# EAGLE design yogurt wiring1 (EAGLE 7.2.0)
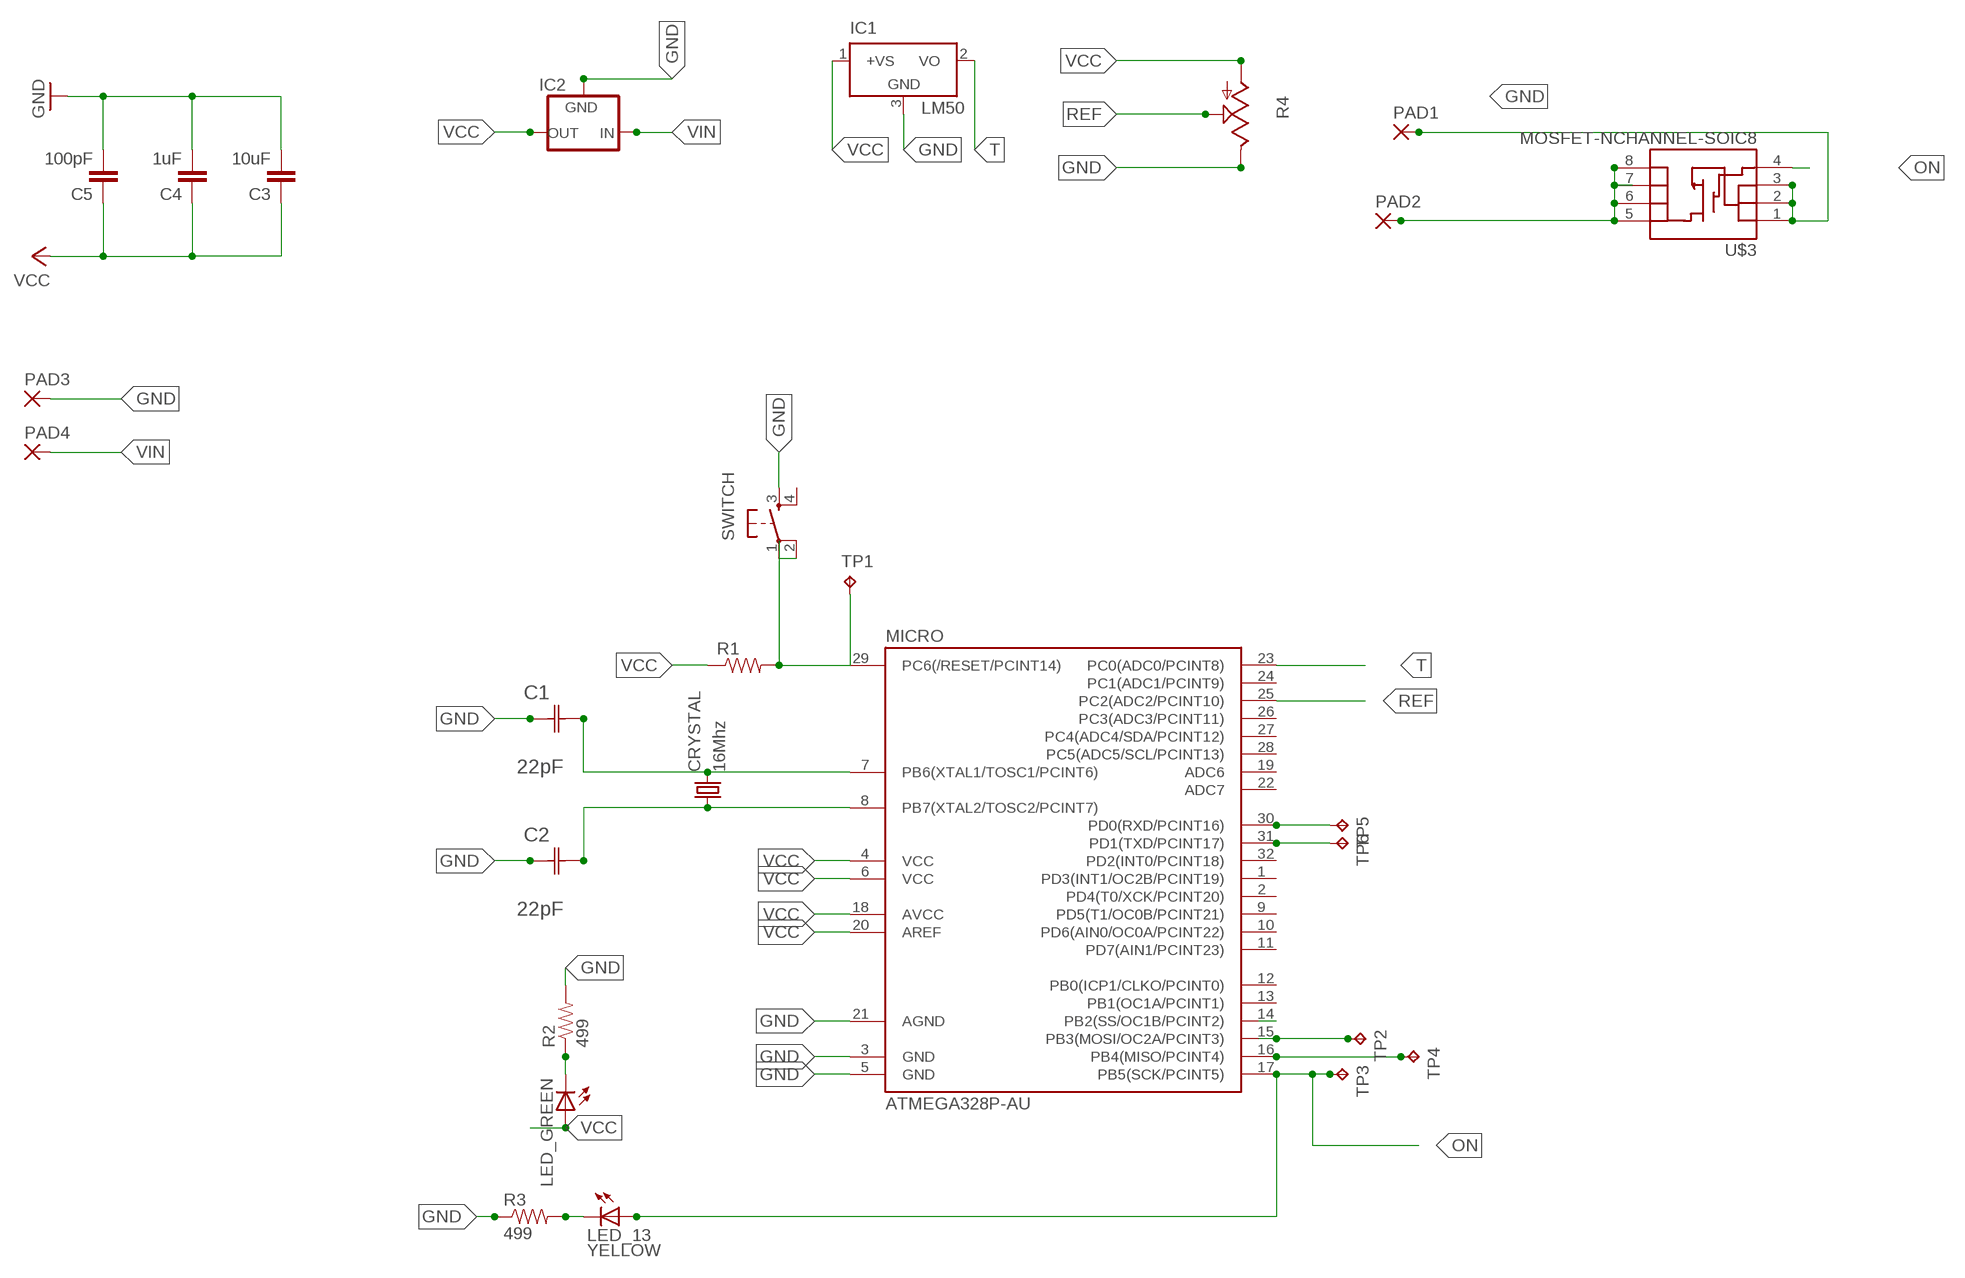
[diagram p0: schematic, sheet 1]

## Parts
C1  22pF  0612ZC225MAT2A  [CAPC3216X178N]
C2  22pF  0612ZC225MAT2A  [CAPC3216X178N]
C3  10uF  CAP1206  [1206]
C4  1uF  CAP1206  [1206]
C5  100pF  CAP1206  [1206]
CRYSTAL  16Mhz  CSM-7X-DU  [CSM-7X-DU]
IC1  LM50  [SOT23]
IC2  V_REG_78XXSIDE  [78XXL]
LED_13  YELLOW  LED1206  [1206]
LED_GREEN  LED1206  [1206]
MICRO  ATMEGA328P-AU  ATMEGA48/88/168-AU  [TQFP32-08]
PAD1  SMD5  [SMD2,54-5,08]
PAD2  SMD5  [SMD2,54-5,08]
PAD3  SMD5  [SMD2,54-5,08]
PAD4  SMD5  [SMD2,54-5,08]
R1  RESISTOR1206  [1206]
R2  499  RESISTOR1206  [1206]
R3  499  RESISTOR1206  [1206]
R4  TRIM_US-SM-42/43X  [SM-42/43X]
SWITCH  6MM_SWITCH6MM_SWITCH  [6MM_SWITCH]
TP1  TPPAD1-17Y  [P1-17Y]
TP2  TPPAD1-17Y  [P1-17Y]
TP3  TPPAD1-17Y  [P1-17Y]
TP4  TPPAD1-17Y  [P1-17Y]
TP5  TPPAD1-17Y  [P1-17Y]
TP6  TPPAD1-17Y  [P1-17Y]
U$3  MOSFET-NCHANNEL-SOIC8  [SO08]

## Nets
GND: C1.1(C1) C2.1(C1) C3.2 C4.2 C5.2 IC1.3(GND) IC2.GND MICRO.3(GND) MICRO.5(GND) MICRO.21(AGND) PAD1.1(P) PAD3.1(P) R2.2 R3.1 R4.3(E) SWITCH.3(S) U$3.1(S) U$3.2(S) U$3.3(S)
N$2: C1.2(C2) CRYSTAL.2 MICRO.7(PB6(XTAL1/TOSC1/PCINT6))
N$4: MICRO.29(PC6(/RESET/PCINT14)) R1.2 SWITCH.1(P) SWITCH.2(P1) TP1.TP
N$5: MICRO.15(PB3(MOSI/OC2A/PCINT3)) TP2.TP
N$6: MICRO.14(PB2(SS/OC1B/PCINT2))
N$7: MICRO.31(PD1(TXD/PCINT17)) TP6.TP
N$8: MICRO.30(PD0(RXD/PCINT16)) TP5.TP
N$9: C2.2(C2) CRYSTAL.1 MICRO.8(PB7(XTAL2/TOSC2/PCINT7))
N$11: MICRO.16(PB4(MISO/PCINT4)) TP4.TP
N$26: LED_GREEN.2(C) R2.1
N$27: LED_13.2(C) R3.2
N$35: PAD2.1(P) U$3.5(D) U$3.6(D) U$3.7(D) U$3.8(D)
ON: LED_13.1(A) MICRO.17(PB5(SCK/PCINT5)) TP3.TP U$3.4(G)
REF: MICRO.25(PC2(ADC2/PCINT10)) R4.2(S)
T: IC1.2(VO) MICRO.23(PC0(ADC0/PCINT8))
VCC: C3.1 C4.1 C5.1 IC1.1(+VS) IC2.OUT LED_GREEN.1(A) MICRO.4(VCC) MICRO.6(VCC) MICRO.18(AVCC) MICRO.20(AREF) R1.1 R4.1(A)
VIN: IC2.IN PAD4.1(P)
Unconnected: MICRO.1(PD3(INT1/OC2B/PCINT19)) MICRO.2(PD4(T0/XCK/PCINT20)) MICRO.9(PD5(T1/OC0B/PCINT21)) MICRO.10(PD6(AIN0/OC0A/PCINT22)) MICRO.11(PD7(AIN1/PCINT23)) MICRO.12(PB0(ICP1/CLKO/PCINT0)) MICRO.13(PB1(OC1A/PCINT1)) MICRO.19(ADC6) MICRO.22(ADC7) MICRO.24(PC1(ADC1/PCINT9)) MICRO.26(PC3(ADC3/PCINT11)) MICRO.27(PC4(ADC4/SDA/PCINT12)) MICRO.28(PC5(ADC5/SCL/PCINT13)) MICRO.32(PD2(INT0/PCINT18)) SWITCH.4(S1)

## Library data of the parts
C1 C2 = AVX_By_element14_Batch_1:0612ZC225MAT2A: Capacitor 1206; MPN: 0612ZC225MAT2A; OC_FARNELL: -; OC_NEWARK: 12N3209; SUPPLIER: AVX; TOLERANCE: ±20%; VALUE: 2.2µF; VOLTAGERATING: 10V
C3-C5 = 01_SparkFun:CAP: Capacitor
CRYSTAL = 01_FAB_Hello:CSM-7X-DU: SMD CRYSTAL; OC_FARNELL: unknown; OC_NEWARK: unknown
IC1 = linear:LM50: SOT-23 Single-Supply Centigrade Temperature Sensor Vout = (10mV/°C x Temp °C) +5mmmV Source: http://cache.national.com/ds/LM/LM50.pdf
IC2 = 01_SparkFun:V_REG_78XX: Voltage Regulator Standard 7805 5V regulator. IGO (Input Ground Output). Spark Fun Electronics SKU : COM-00107
LED_13 LED_GREEN = 01_FAB_Hello:LED
MICRO = atmega8:ATMEGA48/88/168
PAD1-PAD4 = wirepad:SMD5: SMD PAD
R1-R3 = 01_SparkFun:RESISTOR: Resistor
R4 = pot:TRIM_US-: POTENTIOMETER
SWITCH = 01_FAB_Hello:6MM_SWITCH: OMRON SWITCH
TP1-TP6 = testpad:TP: Test pad
U$3 = 01_SparkFun:MOSFET-NCHANNEL-SOIC8: N-Channel MOSFET IRF9410 and NDS8434 are common, SOIC-8 parts.

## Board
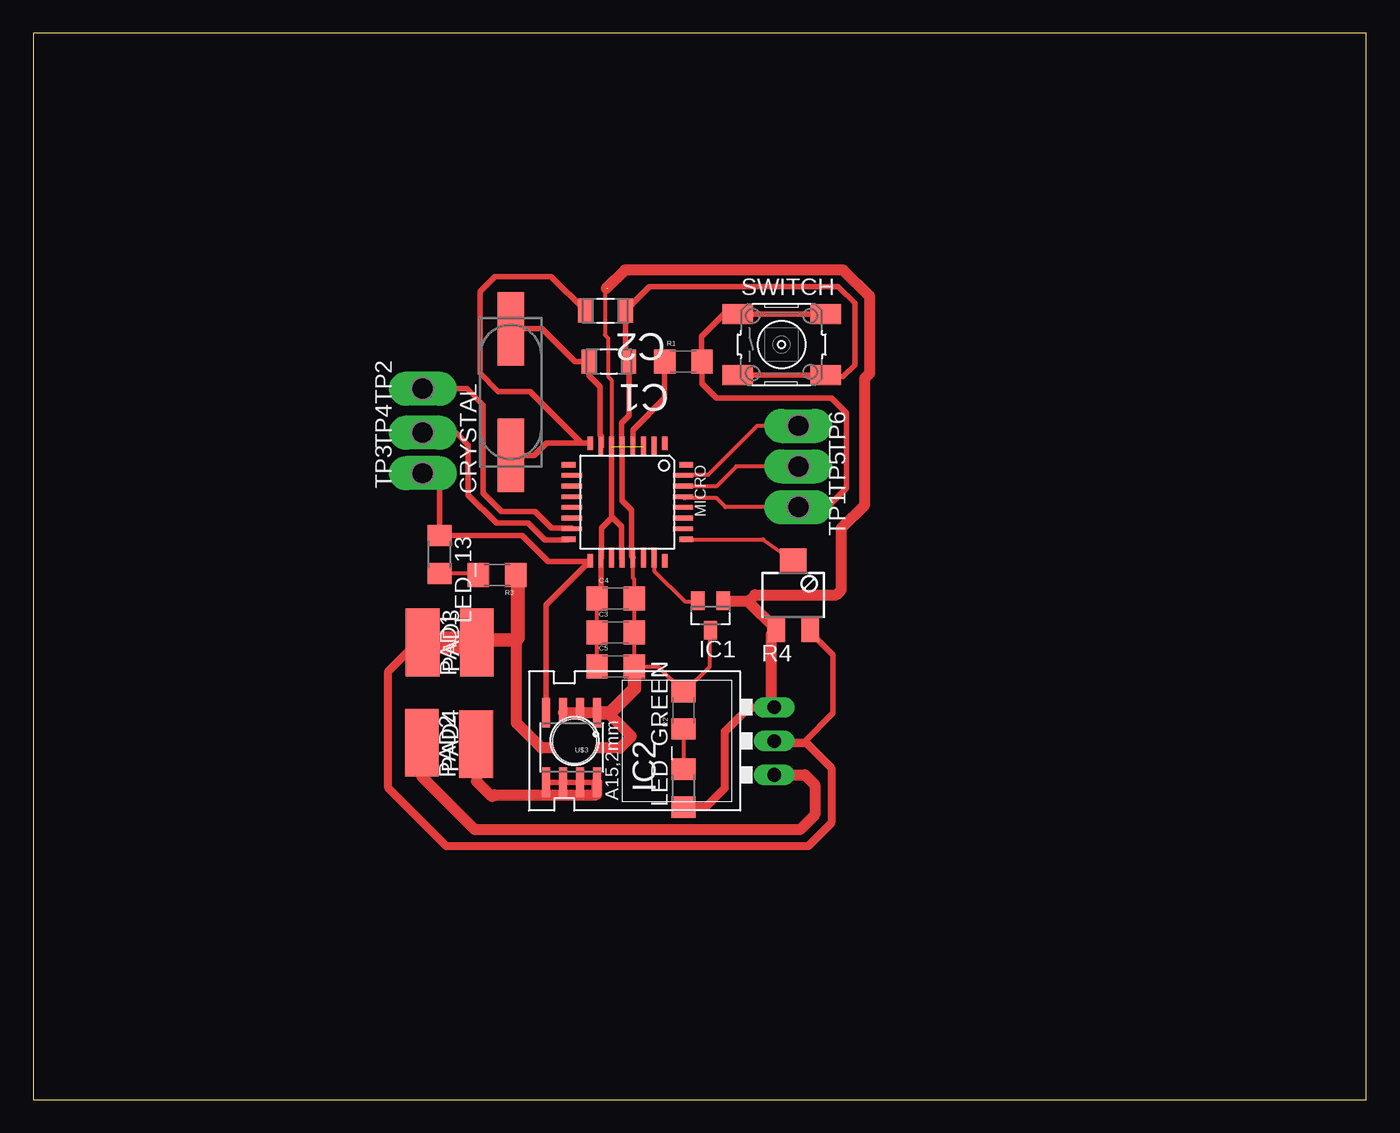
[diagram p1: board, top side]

Size 100 x 80 mm. Coordinates in mm from the lower left corner, seen from the top.
Outline: 0,0 100,0 100,80 0,80 0,0
Copper layers (1*16): Top 0.035mm / dielectric 1.5mm / Bottom 0.035mm
Design rules "default *": minimum track width 16mil, minimum drill 24mil, track to track 12mil, track to pad 12mil, pad to pad 12mil, via to via 12mil, smd to smd 12mil, copper to edge 40mil, drill to drill 8mil, minimum pad ring 10mil, minimum via ring 8mil, stop-mask expansion 4mil, vias tented up to drill 0mil, thermal gap 10mil

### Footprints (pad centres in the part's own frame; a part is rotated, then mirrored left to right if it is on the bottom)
CAPC3216X178N = smd 1.118 x 1.803: 1 -1.499,0; 2 1.499,0
1206 = smd 1.6 x 1.8: 1 -1.4,0; 2 1.4,0
CSM-7X-DU = smd 5.5 x 2: 1 -4.75,0; 2 4.75,0
SOT23 = smd 1 x 1.4: 1 -0.95,-1.1; 2 0.95,-1.1; 3 0,1.1
78XXL = drill 1.016 long: GND 0,-3.81; IN -2.54,-3.81; OUT 2.54,-3.81 | hole 3.302: 0,11.176
1206' = smd 1.6 x 1.803: 1 -1.422,0; 2 1.422,0
TQFP32-08 = smd 1.016 x 0.406: 1 -4.42,2.8; 8 -4.42,-2.8; 17 4.42,-2.8; 24 4.42,2.8 | smd 1.524 x 0.356: 2 -4.166,2; 3 -4.166,1.2; 4 -4.166,0.4; 5 -4.166,-0.4; 6 -4.166,-1.2; 7 -4.166,-2; 18 4.166,-2; 19 4.166,-1.2; 20 4.166,-0.4; 21 4.166,0.4; 22 4.166,1.2; 23 4.166,2 | smd 0.406 x 1.016: 9 -2.8,-4.42; 16 2.8,-4.42; 25 2.8,4.42; 32 -2.8,4.42 | smd 0.356 x 1.524: 10 -2,-4.166; 11 -1.2,-4.166; 12 -0.4,-4.166; 13 0.4,-4.166; 14 1.2,-4.166; 15 2,-4.166; 26 2,4.166; 27 1.2,4.166; 28 0.4,4.166; 29 -0.4,4.166; 30 -1.2,4.166; 31 -2,4.166
SMD2,54-5,08 = smd 2.54 x 5.08: 1 0,0
SM-42/43X = smd 1.3 x 1.9: 1 -1.27,-2.55; 3 1.27,-2.55 | smd 2 x 1.9: 2 0,2.55
6MM_SWITCH = smd 2.286 x 1.524: 1 -3.302,2.286; 2 3.302,2.286; 3 -3.302,-2.286; 4 3.302,-2.286
P1-17Y = drill 1.702 pad 2.121 long: TP 0,0
SO08 = smd 0.61 x 2.21: 1 -1.905,-2.616; 2 -0.635,-2.616; 3 0.635,-2.616; 4 1.905,-2.616; 5 1.905,2.616; 6 0.635,2.616; 7 -0.635,2.616; 8 -1.905,2.616

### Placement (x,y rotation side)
C1  43.18,55.37 180 top
C2  42.93,59.18 180 top
C3  43.69,35.05 0 top
C4  43.69,37.59 0 top
C5  43.69,32.51 0 top
CRYSTAL  35.81,53.09 90 top
IC1  50.8,36.32 180 top
IC2  51.78,26.9 90 top
LED_13  YELLOW  [1206']  30.48,40.89 270 top
LED_GREEN  [1206']  48.77,23.37 90 top
MICRO  44.58,44.83 270 top
PAD1  33.27,34.29 0 top
PAD2  33.21,26.66 0 top
PAD3  29.21,34.29 180 top
PAD4  29.15,26.78 180 top
R1  48.77,55.37 0 top
R2  48.77,29.21 90 top
R3  34.8,39.37 180 top
R4  57.02,37.84 0 top
SWITCH  56.13,56.64 0 top
TP1  57.4,44.45 270 top
TP2  29.21,53.34 90 top
TP3  29.21,46.99 90 top
TP4  29.21,50.04 90 top
TP5  57.4,47.5 270 top
TP6  57.4,50.55 270 top
U$3  40.39,26.42 180 top

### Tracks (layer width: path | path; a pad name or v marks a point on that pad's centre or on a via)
GND  (1 unrouted)
  Top 0.305: MICRO.21 45,40.64 45,39.12 45.09,39.04 C4.2 C3.2 C5.2 46.87,32.51 R2.2 48.86,30.61 50.75,32.5 50.75,35.17 IC1.3
  Top 0.406: MICRO.21 44.88,40.76 44.88,44.25 44.17,44.95 MICRO.5 44.12,49.05 44.12,50.75 44.68,51.3 C1.1 44.42,55.63 C2.1 46.24,61 60.38,61 61.62,59.75 61.62,55.12 60.75,54.25 59.5,54.25 59.39,54.36 SWITCH.3 | R4.3 58.29,35.09 60,33.38 60,29 57.88,26.88 55.61,26.88 IC2.GND | 36.25,39.32 36.38,39.32 36.38,38.25
  Top 0.61: U$3.3 U$3.2 U$3.1 | IC2.GND 55.74,26.75 58,26.75 59.88,24.88 59.88,20.75 58.12,19 31,19 26.62,23.38 26.62,32.12 28.79,34.29 PAD3.1
  Top 0.813: U$3.3 43.09,29.03 44.88,27.25 44,26.38 38.12,26.38 36.25,28.25 36.25,39.32 R3.1
  Top 1.016: PAD1.1 33.48,34.5 36.25,34.5 36.38,34.62 36.38,38.25 36.38,38.75 | C5.2 45.09,30.84 43.25,29 42.32,29 U$3.1
  Top 1.676: PAD3.1 PAD1.1
N$2
  Top 0.406: CRYSTAL.2 38.16,57.84 40.62,55.38 C1.2 41.68,54.32 42.5,53.5 42.5,49.88 42.62,49.75 42.62,49.05 MICRO.7
N$4
  Top 0.305: TP1.TP 51.92,44.45 51.25,45.12 48.84,45.12 MICRO.29
  Top 0.406: SWITCH.2 SWITCH.1 51.8,58.93 50.12,57.25 50.12,55.41 R1.2 50.17,53.71 51.25,52.62 59.88,52.62 61,51.5 61,45.88 59.5,44.38 57.48,44.38 TP1.TP
N$5
  Top 0.406: TP2.TP 32.53,53.34 33.75,52.12 33.75,45.5 35.12,44.12 37.62,44.12 38.88,42.88 40.36,42.88 MICRO.15
N$7
  Top 0.305: TP6.TP 54.3,50.55 50.62,46.88 48.79,46.88 MICRO.31
N$8
  Top 0.305: TP5.TP 52.75,47.5 51.25,46 48.77,46 MICRO.30
N$9
  Top 0.406: CRYSTAL.1 37.59,48.34 38.5,49.25 MICRO.8 41.13,49.25 37.25,53.12 34.88,53.12 33.5,54.5 33.5,60.62 34.62,61.75 38.86,61.75 C2.2
N$11
  Top 0.406: TP4.TP 31.71,50.04 32.62,49.12 32.62,45.38 34.75,43.25 37.12,43.25 38.38,42 40.13,42 MICRO.16
N$26
  Top 0.305: R2.1 LED_GREEN.2
N$27
  Top 0.305: R3.2 33.3,39.47 LED_13.2
N$35
  Top 0.406: U$3.5 U$3.6 U$3.7 U$3.8
  Top 0.813: PAD2.1 33.25,26.62 33.25,23.88 34.38,22.75 34.5,22.75 34.62,22.88 42.25,22.88 42.29,22.92 U$3.8
ON
  Top 0.406: TP3.TP 30.38,47 30.48,46.9 LED_13.1 36.68,42.32 38.62,40.38 41.74,40.38 MICRO.17 38.48,37.12 U$3.4
REF
  Top 0.305: MICRO.25 54.76,42.03 R4.2
T
  Top 0.305: MICRO.23 46.58,39.67 48.88,37.38 49.8,37.38 IC1.2
VCC  (2 unrouted)
  Top 0.305: C5.1 C3.1 C4.1 42.29,38.16 | 44.12,40.61 MICRO.20 | 43.12,60.88 arc90 42.88,60.62 42.88,57.38 43.12,57.12 43.12,54.25 43.38,54 43.38,48.88
  Top 0.406: MICRO.6 43.38,48.88 43.38,43.75 | 43.38,43.75 43.38,43.62 42.62,42.88 42.62,40.71 MICRO.18 42.58,38.16 42.29,38.16 | 44.12,40.61 44.12,43 43.38,43.75 | R1.1 47.37,52.62 45,50.25 45,49.02 MICRO.4
  Top 0.61: LED_GREEN.1 48.82,22 50.5,22 51.88,23.38 51.88,27.62 53.69,29.44 IC2.OUT 55.37,29.66
  Top 0.813: 55.37,29.66 55.37,34.92 R4.1 55.71,35.29 53.62,37.38 51.8,37.38 IC1.1 53.67,37.42 54.12,37.88 60.25,37.88 60.62,38.25 60.62,42.88 62.38,44.62 62.38,54.12 62.75,54.5 62.75,60.25 60.75,62.25 44.38,62.25 43,60.88
VIN
  Top 0.813: IC2.IN 55.61,24.38 57.88,24.38 58.62,23.62 58.62,21.38 57.5,20.25 33.12,20.25 29.15,24.23 PAD4.1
